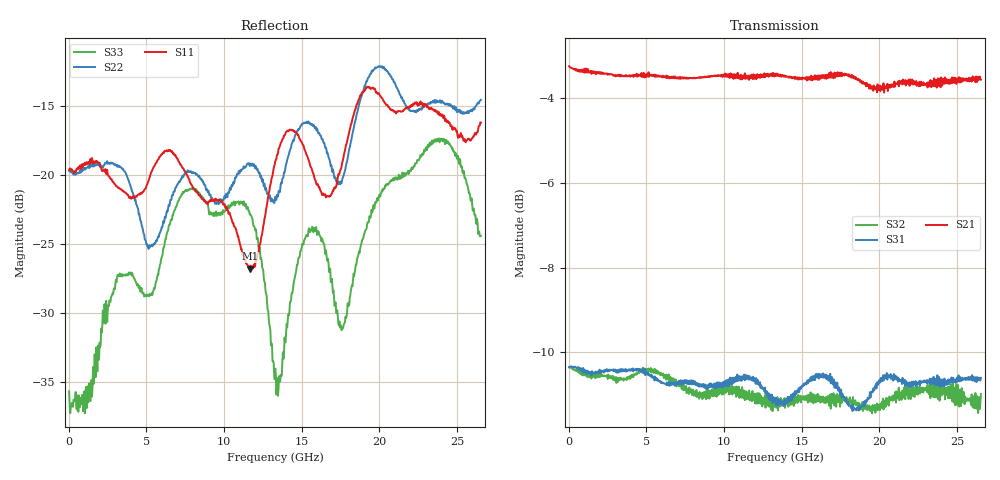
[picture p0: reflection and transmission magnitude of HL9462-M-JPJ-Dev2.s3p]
! 3/13/2020 9:27:10 AM
! H:\PRODUCTION_DATA\TEMP_S3P.S3P
! CHANNEL.1
! TR.MEASUREMENT
! CORRECTED.DATA
# GHZ S RI R 50.0
! FREQ.GHZ  S11RE  S11IM  S12RE  S12IM  S13RE  S13IM
!  S21RE  S21IM  S22RE  S22IM  S23RE  S23IM
!  S31RE  S31IM  S32RE  S32IM  S33RE  S33IM
!; PortSelection: Port_123
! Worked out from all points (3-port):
!   758 points, 35 MHz to 26.53 GHz, reference 50 ohm
!   strongest paths, dB at 35 MHz, 6.65 GHz, 13.3 GHz, 19.91 GHz, 26.53 GHz:
!     S21: -3.2, -3.5, -3.4, -3.8, -3.6
!     S31: -10.4, -10.7, -11.2, -10.8, -10.6
!     S32: -10.4, -10.6, -11.1, -11.3, -11.0
!   lowest |S11| = -26.8 dB at 11.65 GHz (marker M1), VSWR 1.10, Z = 46.8 - j3.1 ohm
!   |S11| at or under -10 dB: start of sweep to end of sweep
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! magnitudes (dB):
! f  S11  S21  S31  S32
! 35 MHz  -19.6  -3.2  -10.4  -10.4
! 5.18 GHz  -20.3  -3.5  -10.5  -10.4
! 7.385 GHz  -19.5  -3.5  -10.8  -10.9
! 11.65 GHz  -26.8  -3.5  -10.6  -11.1
! 13.3 GHz  -19.0  -3.4  -11.2  -11.1
! 15.4 GHz  -18.8  -3.5  -10.7  -11.2
! 17.64 GHz  -19.0  -3.4  -11.0  -11.1
! 19.64 GHz  -13.8  -3.7  -10.9  -11.3
! 23.48 GHz  -15.3  -3.7  -10.6  -10.8
! 26.53 GHz  -16.2  -3.6  -10.6  -11.0
